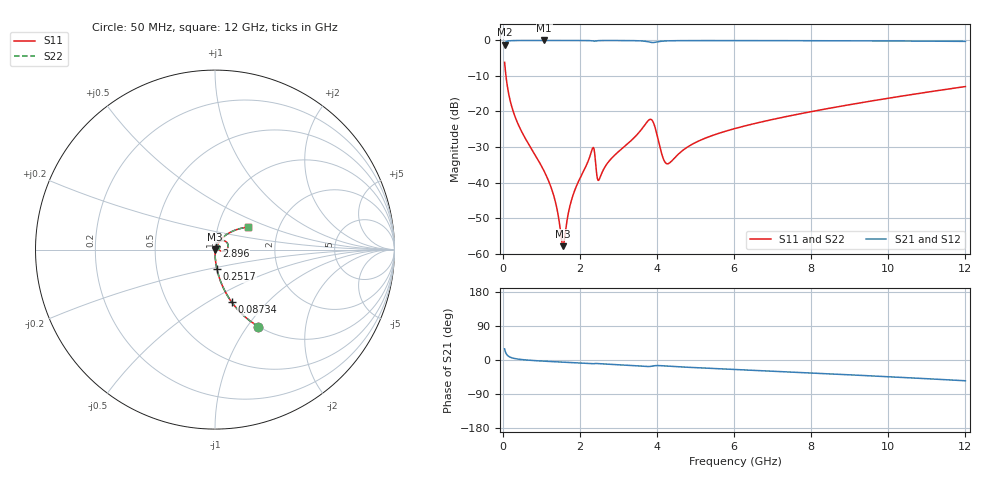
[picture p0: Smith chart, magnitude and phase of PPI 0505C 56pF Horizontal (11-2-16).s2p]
# MHz S MA R 50
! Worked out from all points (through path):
!   1601 points, 50 MHz to 12 GHz, reference 50 ohm
!   highest |S21| = -0.01 dB at 1.073 GHz (marker M1); lowest = -1.2 dB at 50 MHz (marker M2)
!   group delay of S21, straight-line fit = 13.2 ps
!   lowest |S11| = -57.9 dB at 1.566 GHz (marker M3), VSWR 1.00, Z = 50.1 - j0.00917 ohm
!   |S11| at or under -10 dB: 84.75 MHz to end of sweep
!   |S22| runs from -57.9 to -6.2 dB; largest |S21 - S12| = 0
!   S11 on the Smith chart (normalised r, x): 50 MHz: 1.00, -1.13; 87.34 MHz: 1.00, -0.65; 251.7 MHz: 1.00, -0.22; 2.896 GHz: 1.01, +0.05; 12 GHz: 1.40, +0.37
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50  0.4923 -60.7  0.8701 29.3  0.8701 29.3  0.4923 -60.7
87.34375  0.3075 -72.3  0.9512 17.6  0.9512 17.6  0.3075 -72.3
251.6562  0.1091 -84.4  0.9935 5.3  0.9935 5.3  0.1091 -84.4
490.6562  0.0523 -88.0  0.9979 1.2  0.9979 1.2  0.0523 -88.0
1073.219  0.01452 -89.0  0.9988 -3.1  0.9988 -3.1  0.01452 -89.0
1334.625  0.006251 -83.9  0.9987 -4.5  0.9987 -4.5  0.006251 -83.9
1566.156  0.001273 -4.1  0.9986 -5.7  0.9986 -5.7  0.001273 -4.1
1782.75  0.005626 68.4  0.9984 -6.8  0.9984 -6.8  0.005626 68.4
2044.156  0.01268 73.0  0.9979 -8.2  0.9979 -8.2  0.01268 73.0
2320.5  0.02935 52.0  0.9857 -9.9  0.9857 -9.9  0.02935 52.0
2499.75  0.01098 47.0  0.9938 -9.6  0.9938 -9.6  0.01098 47.0
2895.594  0.02404 71.5  0.9968 -11.9  0.9968 -11.9  0.02404 71.5
3806.781  0.07695 31.6  0.9473 -17.1  0.9473 -17.1  0.07695 31.6
3911.344  0.06934 4.3  0.9343 -15.6  0.9343 -15.6  0.06934 4.3
4038.312  0.03893 -13.7  0.9608 -14.7  0.9608 -14.7  0.03893 -13.7
4172.75  0.02117 1.2  0.9794 -15.5  0.9794 -15.5  0.02117 1.2
4284.781  0.01839 26.6  0.9862 -16.3  0.9862 -16.3  0.01839 26.6
4964.438  0.03576 62.3  0.9943 -20.0  0.9943 -20.0  0.03576 62.3
6025  0.05759 61.5  0.9945 -25.0  0.9945 -25.0  0.05759 61.5
8019.156  0.09996 53.6  0.991 -34.4  0.991 -34.4  0.09996 53.6
10013.31  0.154 44.3  0.9835 -44.2  0.9835 -44.2  0.154 44.3
12000  0.2244 34.0  0.9692 -54.8  0.9692 -54.8  0.2244 34.0
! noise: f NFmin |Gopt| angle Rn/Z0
50  0.0003882  0.8643  0.5285  0.0006143
1372  0.004047  0.6784  5.033  0.002427
2701  0.008847  0.7066  9.779  0.005882
4031  0.04074  0.895  14.63  0.08331
5360  0.01467  0.6627  19.15  0.008103
6682  0.01522  0.6114  23.51  0.006982
8012  0.01692  0.5913  27.79  0.007177
9341  0.01894  0.5827  31.94  0.007689
1.067e+04  0.02116  0.5808  35.96  0.008373
1.2e+04  0.02357  0.5836  39.84  0.009206
